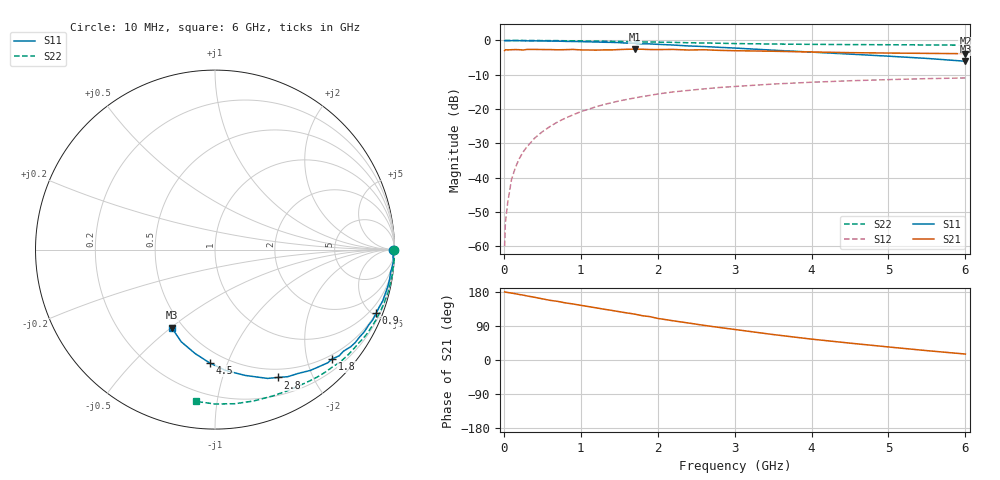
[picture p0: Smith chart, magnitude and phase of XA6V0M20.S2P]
! SIEMENS Discrete & RF Semiconductors
! BFY180
! Si NPN RF Bipolar Junction Transistor in MICRO-X
! VCE = 6 V  IC = 0.2 mA
! Common Emitter S-Parameters:  May  1997
# GHz  S  MA  R  50
!  f  S11  S21  S12  S22
! GHz  MAG  ANG  MAG  ANG  MAG  ANG  MAG  ANG
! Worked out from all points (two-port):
!   36 points, 10 MHz to 6 GHz, reference 50 ohm
!   highest |S21| = -2.53 dB at 1.7 GHz (marker M1); lowest = -3.9 dB at 6 GHz (marker M2)
!   |S21| within 3 dB of the highest: start of sweep to end of sweep
!   lowest |S11| = -6.1 dB at 6 GHz (marker M3), VSWR 2.98, Z = 21.7 - j25.1 ohm
!   |S11| at or under -10 dB: nowhere
!   |S22| runs from -1.4 to 0.0 dB; largest |S21 - S12| = 0.74
!   S11 on the Smith chart (normalised r, x): 10 MHz: open; 900 MHz: 0.50, -5.22; 1.8 GHz: 0.41, -2.48; 2.8 GHz: 0.40, -1.53; 4.5 GHz: 0.41, -0.87; 6 GHz: 0.43, -0.50
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0.01  0.9923 -0.2  0.71 179.8  0.001 75.3  0.9997 -0.1
0.02  0.9895 -0.3  0.733 179.1  0.0022 95.4  0.9999 -0.4
0.05  0.9926 -1.1  0.728 178.2  0.0043 89.0  0.9998 -0.9
0.1  0.993 -2.6  0.733 176.6  0.0094 89.1  0.9999 -2.0
0.15  0.9961 -3.7  0.736 174.8  0.014 88.2  0.9999 -3.0
0.2  0.9929 -4.8  0.733 172.9  0.0188 86.5  0.9986 -4.0
0.3  0.9863 -7.3  0.74 169.1  0.0281 83.7  0.997 -5.9
0.4  0.987 -9.6  0.74 165.5  0.0376 82.2  0.9977 -7.8
0.5  0.9845 -12.1  0.737 161.4  0.0466 79.8  0.9957 -9.8
0.7  0.9771 -17.0  0.731 154.7  0.0649 75.1  0.9933 -13.7
0.9  0.9653 -21.5  0.74 147.8  0.0823 70.7  0.9875 -17.7
1.1  0.9541 -26.1  0.726 141.0  0.0993 66.7  0.9805 -21.5
1.7  0.9102 -40.6  0.747 121.1  0.145 54.6  0.9549 -32.9
1.8  0.8932 -43.0  0.744 116.9  0.152 52.9  0.9523 -34.6
2.2  0.8576 -51.7  0.74 103.5  0.1776 45.1  0.9378 -41.8
2.6  0.8159 -60.2  0.732 91.5  0.1966 38.5  0.9181 -48.2
2.8  0.7941 -63.8  0.717 85.9  0.206 35.3  0.9102 -51.3
3.5  0.7215 -76.4  0.696 67.2  0.2313 25.1  0.8868 -61.5
4  0.676 -85.0  0.679 55.1  0.2458 18.5  0.8767 -68.5
4.5  0.632 -92.7  0.664 44.5  0.2583 12.4  0.8706 -75.6
5.5  0.547 -110.1  0.648 24.7  0.2774 0.8  0.8603 -89.9
6  0.4975 -119.1  0.641 15.7  0.2839 -5.3  0.8525 -97.1
